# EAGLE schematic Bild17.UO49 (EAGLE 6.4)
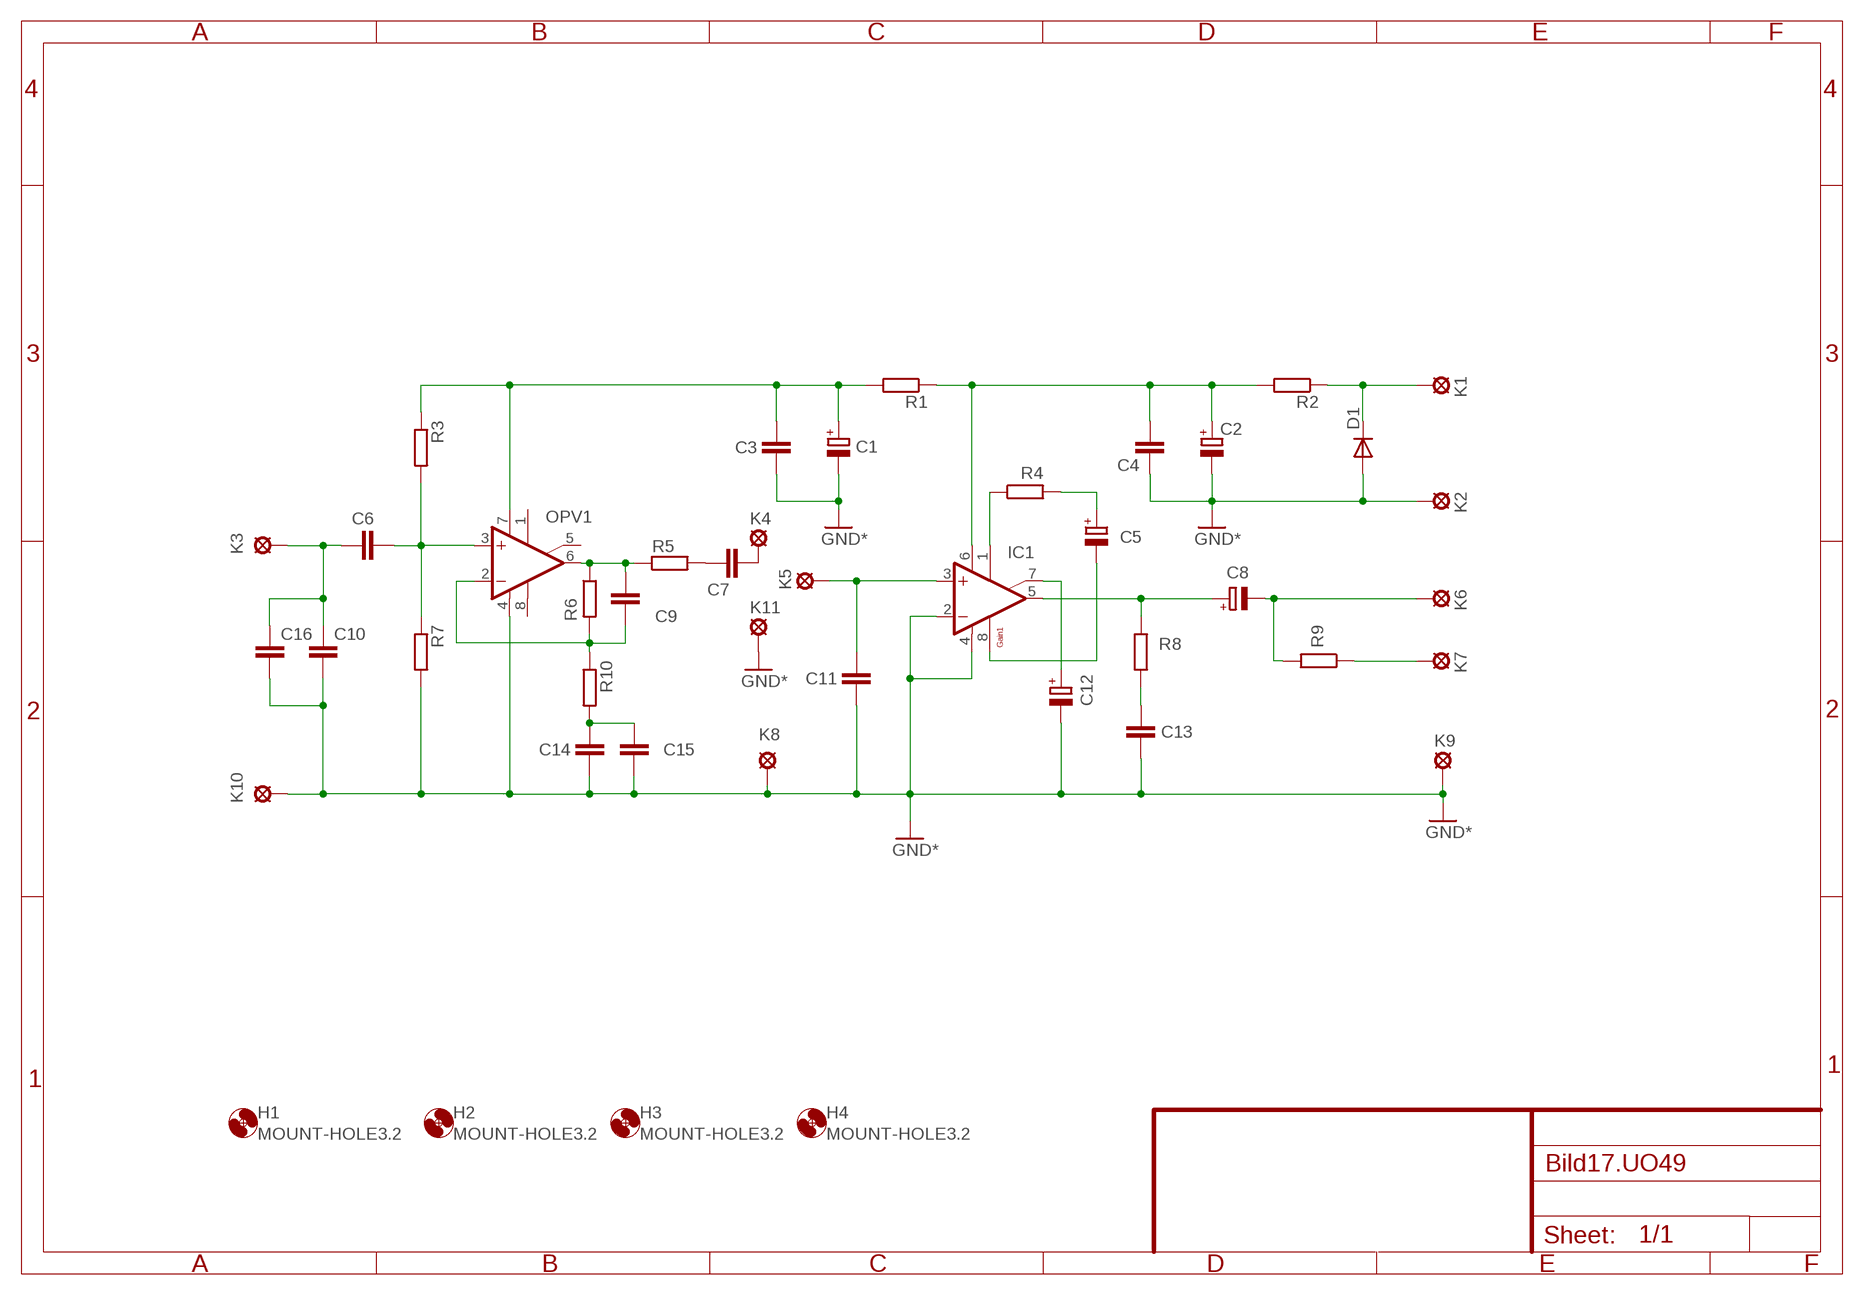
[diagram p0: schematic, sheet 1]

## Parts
C1  CPOL-EUE2-5  [E2-5]
C2  CPOL-EUE5-10.5  [E5-10,5]
C3  C-EU050-035X075  [C050-035X075]
C4  C-EU050-035X075  [C050-035X075]
C5  CPOL-EUE2-5  [E2-5]
C6  C-EU050-035X075  [C050-035X075]
C7  C-EU050-035X075  [C050-035X075]
C8  CPOL-EUE5-10.5  [E5-10,5]
C9  C-EU050-035X075  [C050-035X075]
C10  C-EU050-075X075  [C050-075X075]
C11  C-EU050-035X075  [C050-035X075]
C12  CPOL-EUE2-5  [E2-5]
C13  C-EU050-035X075  [C050-035X075]
C14  C-EU050-050X075  [C050-050X075]
C15  C-EU050-050X075  [C050-050X075]
C16  C-EU050-035X075  [C050-035X075]
D1  1N4004  [DO41-10]
H1  MOUNT-HOLE3.2  [3,2]
H2  MOUNT-HOLE3.2  [3,2]
H3  MOUNT-HOLE3.2  [3,2]
H4  MOUNT-HOLE3.2  [3,2]
IC1  LM386NDIL08  [DIL08]
K1  LSP13  [LSP13]
K2  LSP13  [LSP13]
K3  LSP13  [LSP13]
K4  LSP13  [LSP13]
K5  LSP13  [LSP13]
K6  LSP13  [LSP13]
K7  LSP13  [LSP13]
K8  LSP13  [LSP13]
K9  LSP13  [LSP13]
K10  LSP13  [LSP13]
K11  LSP13  [LSP13]
OPV1  UA741P  [DIL08@1]
R1  R-EU_0207/10E  [0207/10E]
R2  R-EU_0207/10E  [0207/10E]
R3  R-EU_0207/10E  [0207/10E]
R4  R-EU_0207/10E  [0207/10E]
R5  R-EU_0207/10E  [0207/10E]
R6  R-EU_0207/10E  [0207/10E]
R7  R-EU_0207/10E  [0207/10E]
R8  R-EU_0207/10E  [0207/10E]
R9  R-EU_0207/10E  [0207/10E]
R10  R-EU_0207/10E  [0207/10E]

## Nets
GND: C1.- C2.- C3.2 C4.2 C10.1 C11.2 C12.- C13.2 C14.2 C15.2 C16.1 D1.A IC1.2(-IN) IC1.4(GND) K2.MP K8.MP K9.MP K10.MP K11.MP OPV1.4(V-) R7.2 ; supply symbol labelled GND*
N$1: D1.K(C) K1.MP R2.1
N$2: K7.MP R9.1
N$3: C8.+ IC1.5(OUT) R8.1
N$4: C12.+ IC1.7(BYPASS)
N$5: IC1.1(GAIN) R4.1
N$6: C11.1 IC1.3(+IN) K5.MP
N$7: C2.+ C4.1 IC1.6(V+) R1.1 R2.2
N$8: C13.1 R8.2
N$9: C8.- K6.MP R9.2
N$10: C5.+ R4.2
N$11: C5.- IC1.8(GAIN1)
N$13: C1.+ C3.1 OPV1.7(V+) R1.2 R3.1
N$14: C7.1 R5.2
N$15: C7.2 K4.MP
N$16: C14.1 C15.1 R10.2
N$17: C9.2 OPV1.2(-IN) R6.2 R10.1
N$19: C9.1 OPV1.6(OUT) R5.1 R6.1
N$20: C6.2 OPV1.3(+IN) R3.2 R7.1
N$22: C6.1 C10.2 C16.2 K3.MP
Unconnected: OPV1.1(ON1) OPV1.5(ON2) OPV1.8(OPT)

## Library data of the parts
C1 C2 C5 C8 C12 = rcl:CPOL-EU: POLARIZED CAPACITOR, European symbol
C3 C4 C6 C7 C9-C11 C13-C16 = rcl:C-EU: CAPACITOR, European symbol
D1 = diode:1N4004: DIODE
H1-H4 = holes:MOUNT-HOLE: MOUNTING HOLE with drill center marker
IC1 = linear:*386N
K1-K11 = solpad:LSP13: SOLDER PAD
OPV1 = linear:*741P: OP AMP
R1-R10 = rcl:R-EU_: RESISTOR, European symbol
